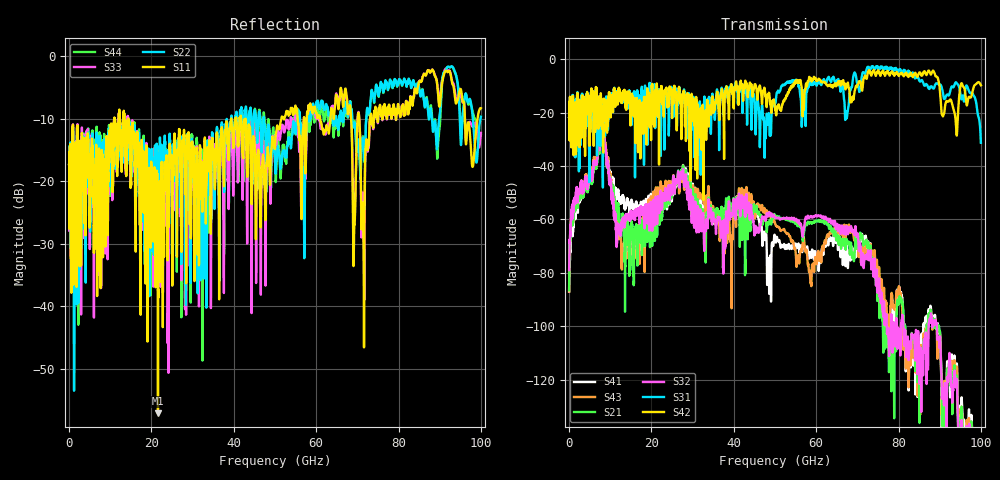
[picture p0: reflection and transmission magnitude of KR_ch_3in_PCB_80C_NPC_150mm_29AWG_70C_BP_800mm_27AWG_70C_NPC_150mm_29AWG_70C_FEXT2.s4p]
# GHz S RI R 45
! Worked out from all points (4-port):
!   4000 points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, 25 MHz to 100 GHz, reference 45 ohm
!   strongest paths, dB at 25 MHz, 25.02 GHz, 50.02 GHz, 75.03 GHz, 100 GHz:
!     S42: -21.8, -20.6, -18.8, -4.2, -9.7
!     S31: -21.7, -16.7, -16.4, -3.0, -31.3
!     S32: -79.0, -48.8, -59.5, -85.9, -150.8
!     S21: -86.5, -49.9, -58.9, -87.8, -153.8
!     S43: -86.9, -47.4, -61.3, -81.4, -144.5
!     S41: -87.1, -51.4, -66.6, -82.9, -144.8
!   lowest |S11| = -57.1 dB at 21.6 GHz (marker M1), VSWR 1.00, Z = 44.9 + j0.0126 ohm
!   |S11| at or under -10 dB: start of sweep to 10.99 GHz; 14.33 GHz to 39.35 GHz (25.01 GHz wide, 93.2 % of centre); 42.85 GHz to 51.56 GHz (8.711 GHz wide, 18.5 % of centre)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
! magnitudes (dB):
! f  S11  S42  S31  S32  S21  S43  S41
! 25 MHz  -17.2  -21.8  -21.7  -79.0  -86.5  -86.9  -87.1
! 8.025 GHz  -16.5  -26.0  -22.9  -27.1  -29.0  -25.7  -27.6
! 13.2 GHz  -9.7  -12.1  -13.5  -59.9  -58.7  -70.9  -51.9
! 21.6 GHz  -57.1  -14.4  -20.0  -51.2  -53.8  -47.9  -50.1
! 27.48 GHz  -14.7  -13.7  -15.9  -44.1  -42.9  -45.3  -42.6
! 77.1 GHz  -9.4  -5.1  -2.8  -97.1  -105.8  -92.2  -97.8
! 100 GHz  -8.3  -9.7  -31.3  -150.8  -153.8  -144.5  -144.8
